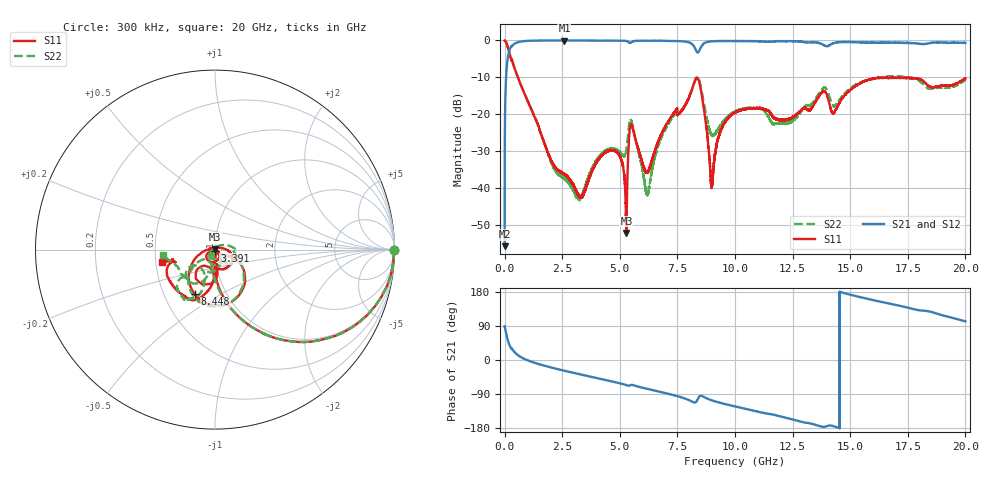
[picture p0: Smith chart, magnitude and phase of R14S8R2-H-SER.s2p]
!{R14S8R2}
!Johanson Technology Inc.
!www.johansontechnology.com
!Test Board Conditions:
!Substrate Type  RO4350B
!Substrate Thickness  20 mil
!Substrate Dk  3.66
!TL Type: GCPW
!TL Trace Width  36 mil
!TL Gap  12 mil
!Electrode orientation  Horizontal
!DUT TOPOLOGY	SERIES
!Mounting Pad LxW  26x36 mil
! Created Wed Nov 25 17:33:21 2020
! 2 Port Network Data from SP1.SP block
! freq  magS11  angS11  magS21  angS21  magS12  angS12  magS22  angS22
# khz S ma R 50
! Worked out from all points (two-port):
!   20001 points, 300 kHz to 20 GHz, reference 50 ohm
!   highest |S21| = -0.01 dB at 2.595 GHz (marker M1); lowest = -55.9 dB at 300 kHz (marker M2)
!   |S21| within 3 dB of the highest: 191.8 MHz to 8.335 GHz (8.143 GHz wide, 191 % of centre); 8.433 GHz to end of sweep
!   lowest |S11| = -52.3 dB at 5.286 GHz (marker M3), VSWR 1.00, Z = 50.1 + j0.213 ohm
!   |S11| at or under -10 dB: 573.5 MHz to end of sweep
!   |S22| runs from -43.4 to 0.0 dB; largest |S21 - S12| = 0.018
!   S11 on the Smith chart (normalised r, x): 300 kHz: open; 3.391 GHz: 0.99, -0.01; 8.448 GHz: 0.71, -0.38; 20 GHz: 0.54, -0.08
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300  0.9972 -0.3  0.001607 89.3  0.001519 89.0  0.9979 -0.2
107300  0.871 -30.4  0.4871 59.6  0.4882 59.4  0.8718 -30.3
255300  0.5935 -55.9  0.8 33.8  0.801 33.8  0.5942 -55.8
837300  0.1979 -85.2  0.9784 3.5  0.9786 3.6  0.1992 -87.0
2595300  0.01557 -31.7  0.9986 -28.3  0.9971 -28.3  0.01329 158.3
3334300  0.007609 -97.0  0.9965 -38.6  0.9968 -38.6  0.007573 -144.9
3391300  0.007799 -110.6  0.9965 -39.4  0.9962 -39.4  0.00815 -136.2
4586300  0.03232 175.7  0.9945 -55.6  0.9945 -55.6  0.03411 -102.8
5015300  0.02646 165.6  0.9933 -61.7  0.9932 -61.7  0.03004 -98.6
5286300  0.002423 61.4  0.9804 -66.4  0.9811 -66.4  0.03225 -60.6
5499300  0.07197 -117.3  0.9405 -65.6  0.9398 -65.7  0.08156 -104.7
6179300  0.01619 -100.7  0.9915 -75.9  0.9932 -75.9  0.008209 139.5
6667300  0.04248 -37.5  0.9925 -82.9  0.9916 -82.9  0.03771 39.3
8153300  0.2256 -42.3  0.8841 -110.3  0.8819 -110.3  0.2244 -44.3
8448300  0.2729 -114.1  0.7226 -96.5  0.7217 -96.3  0.2871 -114.0
8990300  0.01121 89.4  0.9725 -106.4  0.9727 -106.5  0.05186 -108.2
9393300  0.06171 1.0  0.9817 -113.6  0.9807 -113.6  0.07181 -61.4
1.00003e7  0.1046 -22.0  0.9819 -122.4  0.9819 -122.5  0.1077 -46.9
1.22433e7  0.08471 -82.8  0.979 -153.0  0.9806 -152.9  0.07578 -50.8
1.33343e7  0.1221 -84.8  0.9465 -168.3  0.9475 -168.4  0.1363 -106.3
1.66673e7  0.3075 -122.6  0.9326 149.3  0.9256 149.0  0.3248 -119.8
2e7  0.3061 -167.5  0.926 102.1  0.9254 102.3  0.292 -173.6
